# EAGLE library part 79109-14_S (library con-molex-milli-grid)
RECEPTACAL
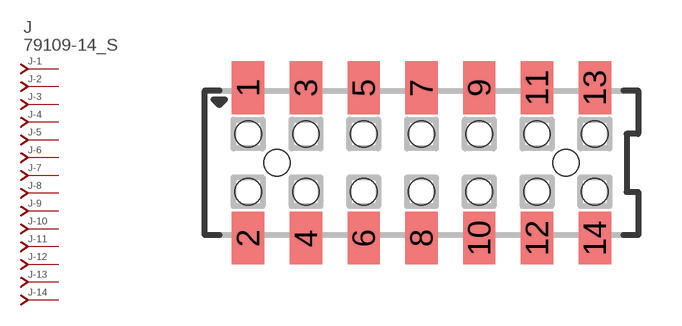
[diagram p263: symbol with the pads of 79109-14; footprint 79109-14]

Designator prefix J; gates -1=J-NV -2=J-N -3=J-N -4=J-N -5=J-N -6=J-N -7=J-N -8=J-N -9=J-N -10=J-N -11=J-N -12=J-N -13=J-N -14=J-N

## 79109-14_S  [79109-14]
1  -1:J  pas
2  -2:J  pas
3  -3:J  pas
4  -4:J  pas
5  -5:J  pas
6  -6:J  pas
7  -7:J  pas
8  -8:J  pas
9  -9:J  pas
10  -10:J  pas
11  -11:J  pas
12  -12:J  pas
13  -13:J  pas
14  -14:J  pas

## Footprint 79109-14 (pad centres in mm)
RECEPTACAL SMD Dual Row, Vertical, Pass-Thru
smd 1.12 x 1.83: 1 -6,2.6; 2 -6,-2.6; 3 -4,2.6; 4 -4,-2.6; 5 -2,2.6; 6 -2,-2.6; 7 0,2.6; 8 0,-2.6; 9 2,2.6; 10 2,-2.6; 11 4,2.6; 12 4,-2.6; 13 6,2.6; 14 6,-2.6
hole 0.914 at -5,0
hole 0.914 at -6,1
hole 0.914 at -6,-1
hole 0.914 at -4,-1
hole 0.914 at -4,1
hole 0.914 at -2,-1
hole 0.914 at -2,1
hole 0.914 at 5,0
hole 0.914 at 0,1
hole 0.914 at 0,-1
hole 0.914 at 2,1
hole 0.914 at 2,-1
hole 0.914 at 4,1
hole 0.914 at 4,-1
hole 0.914 at 6,1
hole 0.914 at 6,-1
